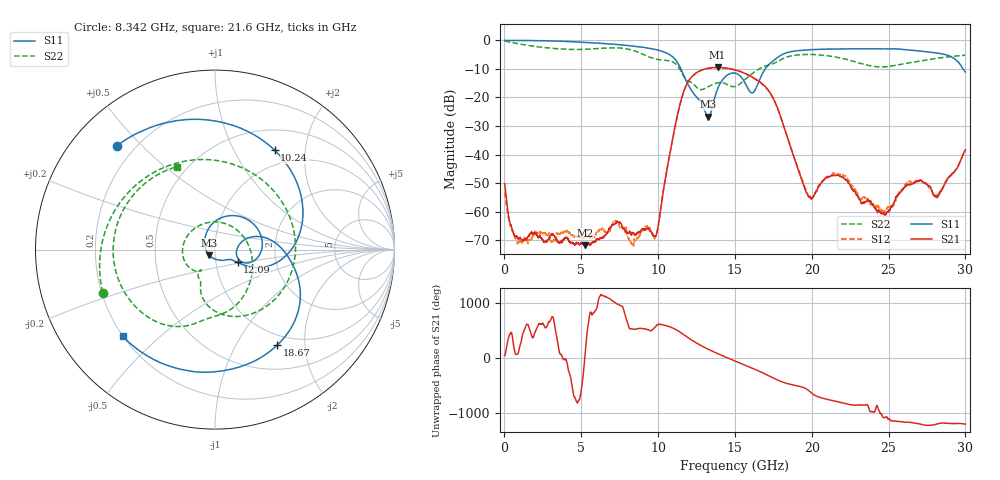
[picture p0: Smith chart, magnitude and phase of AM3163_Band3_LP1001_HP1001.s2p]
!Agilent Technologies,E8364B,MY43040894,A.07.50.67
!Agilent E8364B: A.07.50.67
!Date: Thursday, August 20, 2020 11:07:57
!Correction: S11(Full 2 Port(1,2))
!S21(Full 2 Port(1,2))
!S12(Full 2 Port(1,2))
!S22(Full 2 Port(1,2))
!S2P File: Measurements: S11, S21, S12, S22:
# Hz S  dB  R 50
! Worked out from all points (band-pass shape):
!   3201 points, 10 MHz to 30 GHz, reference 50 ohm
!   highest |S21| = -9.47 dB at 13.87 GHz (marker M1); lowest = -71.8 dB at 5.221 GHz (marker M2)
!   |S21| within 3 dB of the highest: 12.24 GHz to 15.99 GHz (3.751 GHz wide, 26.6 % of centre)
!   lowest |S11| = -26.8 dB at 13.26 GHz (marker M3), VSWR 1.10, Z = 46.7 - j3.01 ohm
!   |S11| at or under -10 dB: 11.48 GHz to 16.97 GHz (5.487 GHz wide, 38.6 % of centre); 29.85 GHz to end of sweep
!   |S22| runs from -17.3 to -0.2 dB; largest |S21 - S12| = 0.0065
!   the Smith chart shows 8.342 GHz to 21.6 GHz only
!   S11 on the Smith chart (normalised r, x): 8.342 GHz: 0.13, +0.42; 10.24 GHz: 0.78, +1.47; 12.09 GHz: 1.27, -0.18; 18.67 GHz: 0.84, -1.50; 21.6 GHz: 0.20, -0.38
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1e7  -0.03 -2.0  -50.21 46.5  -53.22 143.2  -0.22 -6.1
1.097138e9  -0.05 -29.8  -69.75 -50.6  -70.29 -88.0  -1.39 -84.5
2.437316e9  -0.13 -66.0  -69.51 -99.2  -67.43 56.5  -2.43 -166.8
5.014581e9  -0.63 -133.6  -71.16 157.0  -68.72 -115.1  -3.16 57.0
5.220762e9  -0.69 -139.0  -71.82 -20.8  -68.74 -123.6  -3.13 45.7
7.188856e9  -1.39 168.1  -64.27 -63.5  -63.07 -57.9  -2.61 -73.7
8.341597e9  -1.97 133.5  -67.53 174.5  -71.79 164.6  -3.48 -159.1
9.250669e9  -2.61 101.9  -66.26 169.5  -65.17 177.4  -5.43 119.3
1.000979e10  -3.43 70.3  -65.07 -98.0  -65.01 -136.8  -6.73 41.5
1.024409e10  -3.80 59.0  -56.63 -107.6  -55.97 -105.4  -6.89 17.1
1.209035e10  -16.83 -29.4  -13.38 -10.6  -13.47 -10.1  -14.52 -117.6
1.326183e10  -26.78 -135.4  -9.77 166.2  -9.81 166.4  -16.24 -127.7
1.3871e10  -17.02 97.7  -9.47 87.1  -9.58 87.4  -14.90 -154.8
1.5005e10  -11.49 8.1  -10.35 -48.3  -10.32 -47.5  -16.19 72.4
1.6139e10  -18.40 -3.5  -12.91 179.1  -13.00 178.9  -11.58 -41.5
1.721676e10  -8.43 -0.4  -17.77 40.7  -17.93 42.1  -8.61 -89.8
1.86694e10  -3.94 -57.1  -38.22 -117.3  -38.08 -114.3  -5.44 -137.5
2.000958e10  -3.24 -98.0  -55.45 83.3  -55.15 83.3  -4.94 174.4
2.16028e10  -3.03 -136.7  -47.25 -64.5  -46.80 -65.9  -5.87 114.7
2.500479e10  -3.01 145.3  -59.46 -29.3  -58.35 -115.3  -9.16 -63.1
2.735713e10  -3.93 80.0  -49.97 -137.3  -49.98 -127.7  -6.95 -165.2
3e10  -11.11 -23.7  -38.38 -117.5  -38.42 -118.3  -5.18 110.3
